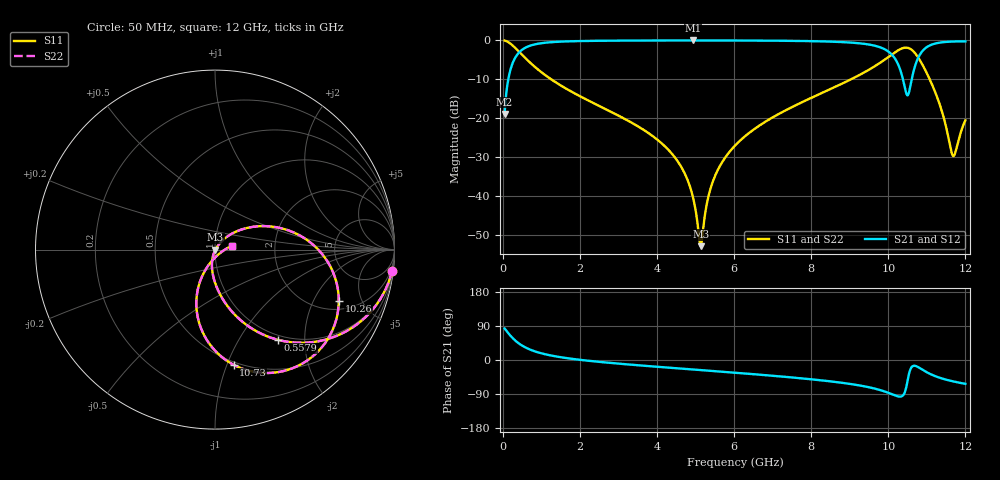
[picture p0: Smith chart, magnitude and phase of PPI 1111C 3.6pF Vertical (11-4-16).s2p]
# GHz S MA R 50
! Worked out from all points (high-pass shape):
!   1601 points, 50 MHz to 12 GHz, reference 50 ohm
!   highest |S21| = -0.02 dB at 4.935 GHz (marker M1); lowest = -18.9 dB at 50 MHz (marker M2)
!   |S21| within 3 dB of the highest: 433.3 MHz to 10.02 GHz (9.589 GHz wide, 183 % of centre); 10.86 GHz to end of sweep
!   lowest |S11| = -52.8 dB at 5.136 GHz (marker M3), VSWR 1.00, Z = 50.2 - j0.0959 ohm
!   |S11| at or under -10 dB: 1.258 GHz to 9.033 GHz (7.775 GHz wide, 151 % of centre); 11.07 GHz to end of sweep
!   |S22| runs from -52.8 to -0.1 dB; largest |S21 - S12| = 0
!   S11 on the Smith chart (normalised r, x): 50 MHz: 1, -17; 557.9 MHz: 0.93, -1.49; 10.26 GHz: 2.48, -3.21; 10.73 GHz: 0.48, -1.06; 12 GHz: 1.20, +0.05
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0.05  0.9935 -6.8  0.1139 83.2  0.1139 83.2  0.9935 -6.8
0.2367188  0.8784 -29.8  0.4776 60.2  0.4776 60.2  0.8784 -29.8
0.557875  0.6127 -55.1  0.7897 34.8  0.7897 34.8  0.6127 -55.1
1.080688  0.365 -74.2  0.93 15.7  0.93 15.7  0.365 -74.2
2.044156  0.1874 -89.6  0.9809 0.0  0.9809 0.0  0.1874 -89.6
4.038312  0.05178 -106.0  0.9965 -18.1  0.9965 -18.1  0.05178 -106.0
4.605937  0.02491 -107.8  0.9973 -22.6  0.9973 -22.6  0.02491 -107.8
4.934563  0.009699 -102.0  0.9975 -25.1  0.9975 -25.1  0.009699 -102.0
5.136219  0.00228 -24.8  0.9974 -26.6  0.9974 -26.6  0.00228 -24.8
5.315469  0.008968 46.8  0.9973 -28.0  0.9973 -28.0  0.008968 46.8
5.457375  0.01574 52.0  0.9971 -29.1  0.9971 -29.1  0.01574 52.0
6.025  0.04456 53.0  0.9959 -33.6  0.9959 -33.6  0.04456 53.0
8.019156  0.1844 37.3  0.9771 -51.1  0.9771 -51.1  0.1844 37.3
9.408344  0.3959 17.1  0.8981 -70.0  0.8981 -70.0  0.3959 17.1
10.01331  0.6159 -4.4  0.712 -87.0  0.712 -87.0  0.6159 -4.4
10.25978  0.7467 -22.6  0.4864 -96.2  0.4864 -96.2  0.7467 -22.6
10.49878  0.8035 -50.4  0.1966 -55.8  0.1966 -55.8  0.8035 -50.4
10.73031  0.6499 -80.8  0.528 -16.6  0.528 -16.6  0.6499 -80.8
10.94691  0.4273 -101.5  0.782 -29.3  0.782 -29.3  0.4273 -101.5
11.27553  0.1817 -115.5  0.9246 -44.8  0.9246 -44.8  0.1817 -115.5
11.67137  0.03325 -59.9  0.9662 -56.2  0.9662 -56.2  0.03325 -59.9
12  0.09419 12.4  0.9713 -62.9  0.9713 -62.9  0.09419 12.4
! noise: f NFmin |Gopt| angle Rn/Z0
0.05  0.0004764  0.9134  2.806  0.001212
1.372  0.003828  0.6805  8.572  0.002306
2.701  0.006268  0.6299  15.04  0.003127
4.031  0.008549  0.6068  21.45  0.003892
5.36  0.01096  0.6019  27.66  0.004805
6.682  0.01398  0.6174  33.61  0.006266
8.012  0.0194  0.6693  39.54  0.01004
9.341  0.03884  0.7995  45.82  0.03412
10.67  0.2687  0.9651  52.22  1.405
12  0.04735  0.8034  57.53  0.03857
